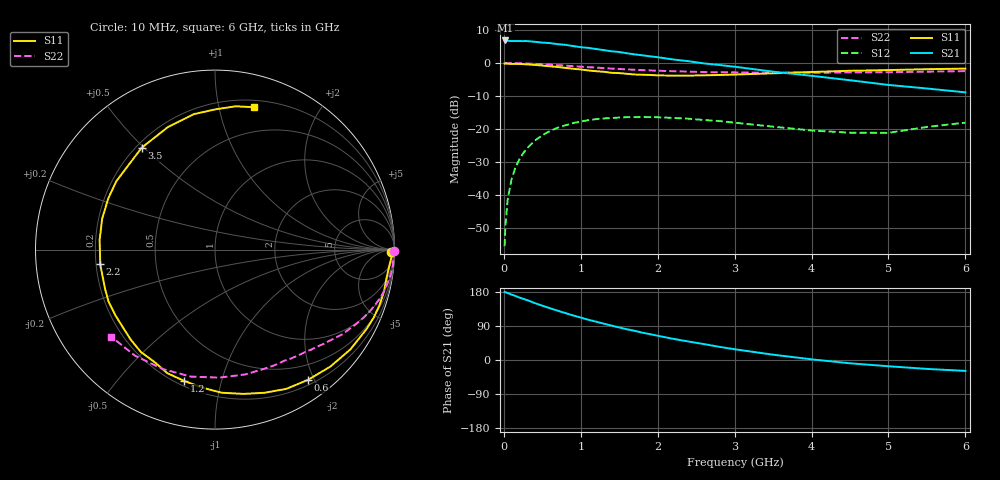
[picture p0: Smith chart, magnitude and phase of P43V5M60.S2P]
! SIEMENS Small Signal Semiconductors
! BFP182
! Si NPN RF Bipolar Junction Transistor in SOT143
! VCE = 3.5 V  IC = 0.6 mA
! Common Emitter S-Parameters:  March  1996
# GHz  S  MA  R  50
!  f  S11  S21  S12  S22
! GHz  MAG  ANG  MAG  ANG  MAG  ANG  MAG  ANG
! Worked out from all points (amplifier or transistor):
!   36 points, 10 MHz to 6 GHz, reference 50 ohm
!   highest |S21| = 6.8 dB at 20 MHz (marker M1)
!   |S21| within 3 dB of that: start of sweep to 1.322 GHz
!   unconditionally stable (mu >= 1): 2.897 GHz to end of sweep
!   at 250 MHz: K = 0.08, MSG = 17.0 dB, |S12| = -27.4 dB
!   at 1.4 GHz: K = 0.50, MSG = 10.1 dB, |S12| = -16.6 dB
!   at 6 GHz: K = 1.18, MAG = 2.0 dB, |S12| = -18.0 dB
!   S11 on the Smith chart (normalised r, x): 10 MHz: 62, -51; 600 MHz: 0.27, -1.92; 1.2 GHz: 0.23, -0.77; 2.2 GHz: 0.22, -0.06; 3.5 GHz: 0.22, +0.49; 6 GHz: 0.26, +1.28
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0.01  0.9809 -0.9  2.16 179.7  0.0017 81.2  0.9989 -0.3
0.02  0.986 -1.9  2.194 179.2  0.0034 87.2  0.9931 -0.7
0.05  0.9772 -4.6  2.168 176.5  0.0087 89.5  0.9972 -1.7
0.1  0.9691 -9.1  2.148 172.7  0.0173 84.0  0.9948 -3.3
0.15  0.9699 -14.0  2.148 169.0  0.0262 80.7  0.995 -5.1
0.3  0.9533 -27.7  2.149 158.3  0.0511 72.3  0.9827 -10.0
0.4  0.937 -36.4  2.095 150.4  0.0667 66.5  0.973 -13.2
0.6  0.8919 -54.4  2.002 136.6  0.0938 55.2  0.9438 -19.1
0.8  0.8438 -71.0  1.883 123.8  0.1144 45.0  0.9117 -24.4
1.1  0.772 -95.3  1.694 106.1  0.137 32.1  0.8654 -31.3
1.2  0.7516 -103.2  1.627 101.1  0.1418 27.6  0.8525 -33.6
1.4  0.7116 -118.2  1.505 90.8  0.1476 20.6  0.8242 -37.3
1.6  0.6871 -133.1  1.404 81.1  0.1518 14.4  0.8023 -40.9
1.8  0.6647 -146.8  1.308 72.2  0.1524 9.0  0.7818 -44.1
2.2  0.6446 -172.7  1.132 55.9  0.1479 -0.5  0.7523 -51.1
2.8  0.6596 154.3  0.934 34.8  0.1326 -10.4  0.7258 -61.8
3.5  0.6992 125.8  0.74 14.0  0.109 -14.5  0.7157 -76.4
4  0.7314 111.0  0.641 1.8  0.0953 -10.6  0.7137 -88.1
4.5  0.7639 98.8  0.549 -8.7  0.0884 -3.5  0.7203 -100.8
5  0.7818 89.7  0.466 -16.5  0.088 9.6  0.7264 -113.7
5.5  0.8069 81.7  0.412 -23.5  0.1079 14.9  0.7405 -127.1
6  0.823 74.5  0.36 -28.8  0.1255 15.5  0.7547 -140.0
